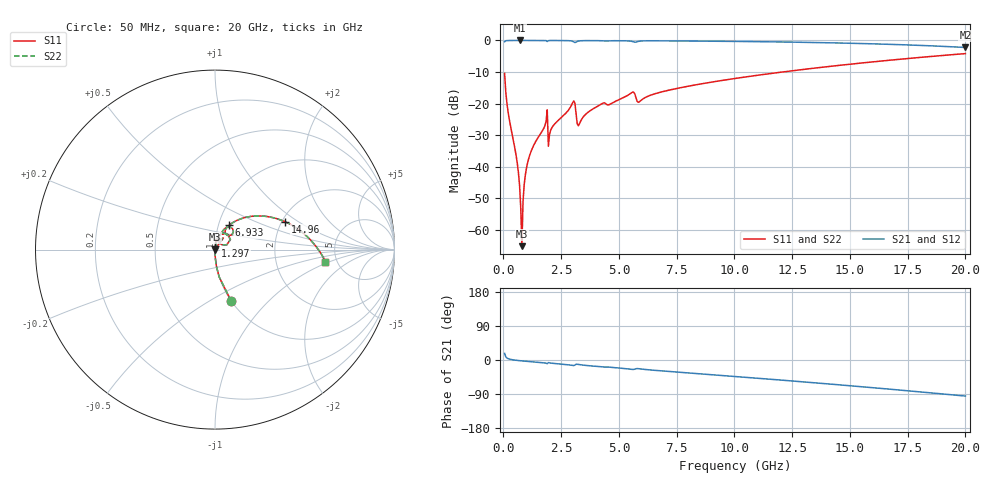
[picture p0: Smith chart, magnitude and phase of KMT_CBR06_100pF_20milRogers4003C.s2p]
! Data measured by Modelithics Inc. support@modelithics.com 813-866-6335
! KEMET CBR0603 100pF, Pad Width= 0.851mm, Pad Length= 0.64mm, Pad Gap= 0.62mm, 20mil Rogers 4003C substrate Data, January 2022
# hz S ma R 50
! 2 Port Network Data from SP1.SP block
! freq  magS11  angS11  magS21  angS21  magS12  angS12  magS22  angS22
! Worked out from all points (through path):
!   401 points, 50 MHz to 20 GHz, reference 50 ohm
!   highest |S21| = 0.00 dB at 698.4 MHz (marker M1); lowest = -2.2 dB at 20 GHz (marker M2)
!   group delay of S21, straight-line fit = 13.3 ps
!   lowest |S11| = -65.1 dB at 798.1 MHz (marker M3), VSWR 1.00, Z = 50 + j0.0348 ohm
!   |S11| at or under -10 dB: start of sweep to 12.06 GHz
!   |S22| runs from -65.1 to -4.2 dB; largest |S21 - S12| = 0
!   S11 on the Smith chart (normalised r, x): 50 MHz: 1.00, -0.63; 1.297 GHz: 1.00, +0.04; 6.933 GHz: 1.12, +0.31; 14.96 GHz: 2.07, +0.78; 20 GHz: 4.05, -0.88
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5e7  0.3014 -72.5  0.9532 17.4  0.9532 17.4  0.3014 -72.5
5.98625e8  0.01139 -89.3  0.9996 -1.1  0.9996 -1.1  0.01139 -89.3
6.98375e8  0.005062 -87.3  0.9996 -1.8  0.9996 -1.8  0.005062 -87.3
7.98125e8  0.0005546 38.8  0.9996 -2.4  0.9996 -2.4  0.0005546 38.8
8.97875e8  0.005188 82.2  0.9995 -2.9  0.9995 -2.9  0.005188 82.2
9.4775e8  0.007422 83.3  0.9995 -3.2  0.9995 -3.2  0.007422 83.3
1.0475e9  0.01166 83.9  0.9994 -3.7  0.9994 -3.7  0.01166 83.9
1.296875e9  0.02141 83.5  0.9992 -5.0  0.9992 -5.0  0.02141 83.5
1.795625e9  0.04475 80.1  0.9973 -7.8  0.9973 -7.8  0.04475 80.1
2.045e9  0.03803 79.6  0.9977 -8.2  0.9977 -8.2  0.03803 79.6
2.992625e9  0.1028 61.8  0.9705 -14.5  0.9705 -14.5  0.1028 61.8
3.242e9  0.04467 50.2  0.9781 -11.7  0.9781 -11.7  0.04467 50.2
3.391625e9  0.05689 69.2  0.9907 -13.1  0.9907 -13.1  0.05689 69.2
5.53625e9  0.148 58.5  0.9711 -24.6  0.9711 -24.6  0.148 58.5
5.885375e9  0.107 56.1  0.9744 -23.2  0.9744 -23.2  0.107 56.1
6.73325e9  0.1494 60.8  0.9859 -28.2  0.9859 -28.2  0.1494 60.8
6.93275e9  0.156 60.0  0.9851 -29.1  0.9851 -29.1  0.156 60.0
1.0025e10  0.2502 46.1  0.9658 -43.5  0.9658 -43.5  0.2502 46.1
1.336662e10  0.3611 29.9  0.9292 -59.6  0.9292 -59.6  0.3611 29.9
1.496262e10  0.4191 21.8  0.9039 -67.7  0.9039 -67.7  0.4191 21.8
1.670825e10  0.486 12.6  0.8686 -76.9  0.8686 -76.9  0.486 12.6
2e10  0.619 -6.2  0.7739 -95.2  0.7739 -95.2  0.619 -6.2
